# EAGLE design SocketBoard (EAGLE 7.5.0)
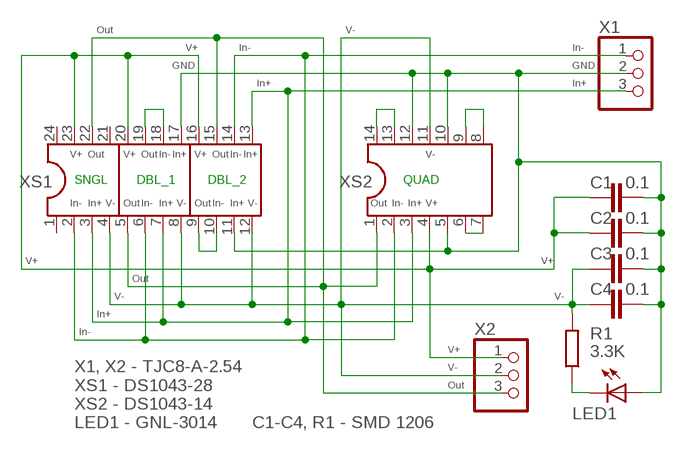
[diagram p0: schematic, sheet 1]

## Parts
C1  0.1  C-EUC1206  [C1206]
C2  0.1  C-EUC1206  [C1206]
C3  0.1  C-EUC1206  [C1206]
C4  0.1  C-EUC1206  [C1206]
LED1  GNL-3014  LED3MM  [LED3MM]
R1  3.3K  R-EU_R1206  [R1206]
X1  KF2510  PINHD-1X3  [1X03]
X2  KF2510  PINHD-1X3  [1X03]
XS1  DS1043-28  DIL24-3  [DIL24-3]
XS2  DS1043-14  DIL14  [DIL14]

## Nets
GND: C1.2 C2.2 C3.1 C4.1 LED1.A X1.2 XS1.11 XS1.17 XS2.5 XS2.10 XS2.12
IN+: X1.3 XS1.3 XS1.7 XS1.13 XS2.3
IN-: X1.1 XS1.2 XS1.6 XS1.14 XS2.2
N$1: XS1.9 XS1.10
N$2: XS1.18 XS1.19
N$3: XS2.13 XS2.14
N$4: XS2.8 XS2.9
N$5: XS2.6 XS2.7
N$8: LED1.K(C) R1.1
OUT: X2.3 XS1.5 XS1.15 XS1.22 XS2.1
V+: C1.1 C2.1 X2.1 XS1.16 XS1.20 XS1.23 XS2.4
V-: C3.2 C4.2 R1.2 X2.2 XS1.4 XS1.8 XS1.12 XS2.11
Unconnected: XS1.1 XS1.21 XS1.24

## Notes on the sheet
- Out | V-
- V+ | In- | In-
- GND | GND
- In+ | In+
- V+ | Out | V+ | Out | In- | In+ | V+ | Out | In- | In+ | V-
- SNGL | DBL_1 | DBL_2 | QUAD
- In- | In+ | V- | Out | In- | In+ | V- | Out | In- | In+ | V- | Out | In- | In+ | V+
- V+ | V+
- Out
- V- | V-
- In+
- In-
- V+
- V-
- Out
- X1, X2 - TJC8-A-2.54
  XS1 - DS1043-28
  XS2 - DS1043-14
  LED1 - GNL-3014
- C1-C4, R1 - SMD 1206

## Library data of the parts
C1-C4 = resistor:C-EU: CAPACITOR, European symbol
LED1 = led:LED: LED
R1 = resistor:R-EU_: RESISTOR, European symbol
X1 X2 = pinhead:PINHD-1X3: PIN HEADER
XS1 = ic-package:DIL24: Dual In Line
XS2 = ic-package:DIL14: Dual In Line / Socket

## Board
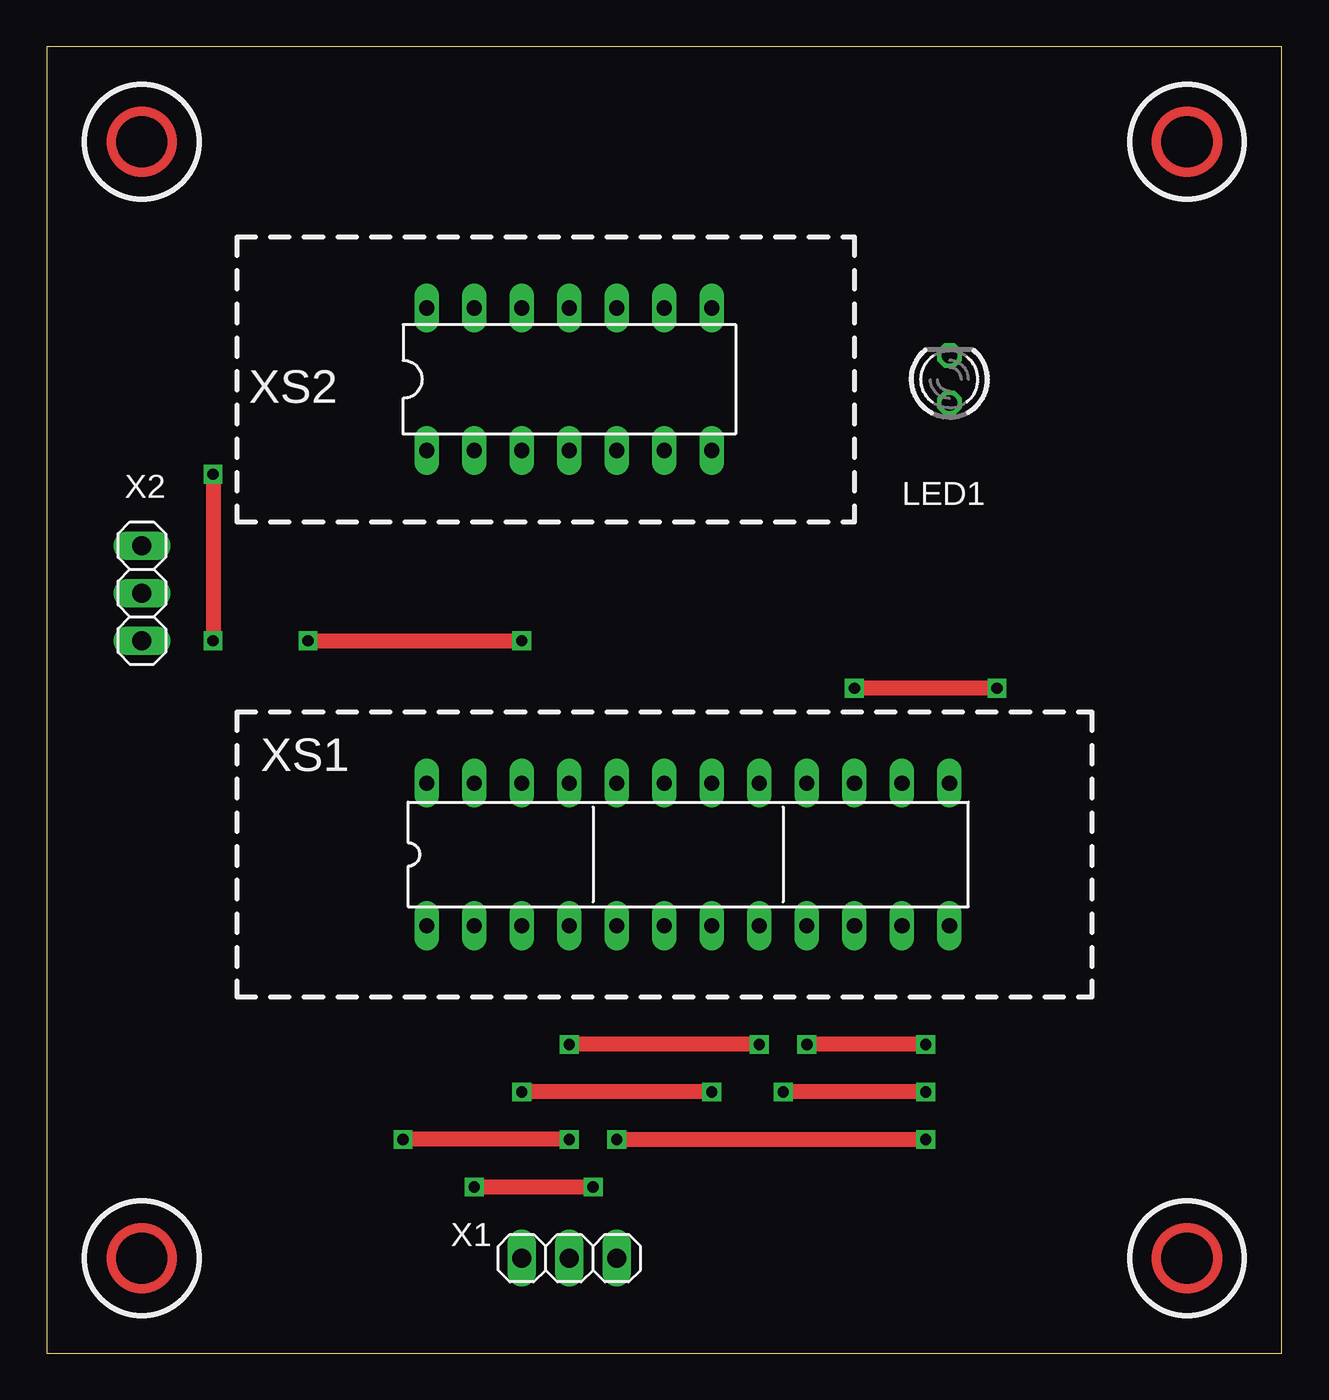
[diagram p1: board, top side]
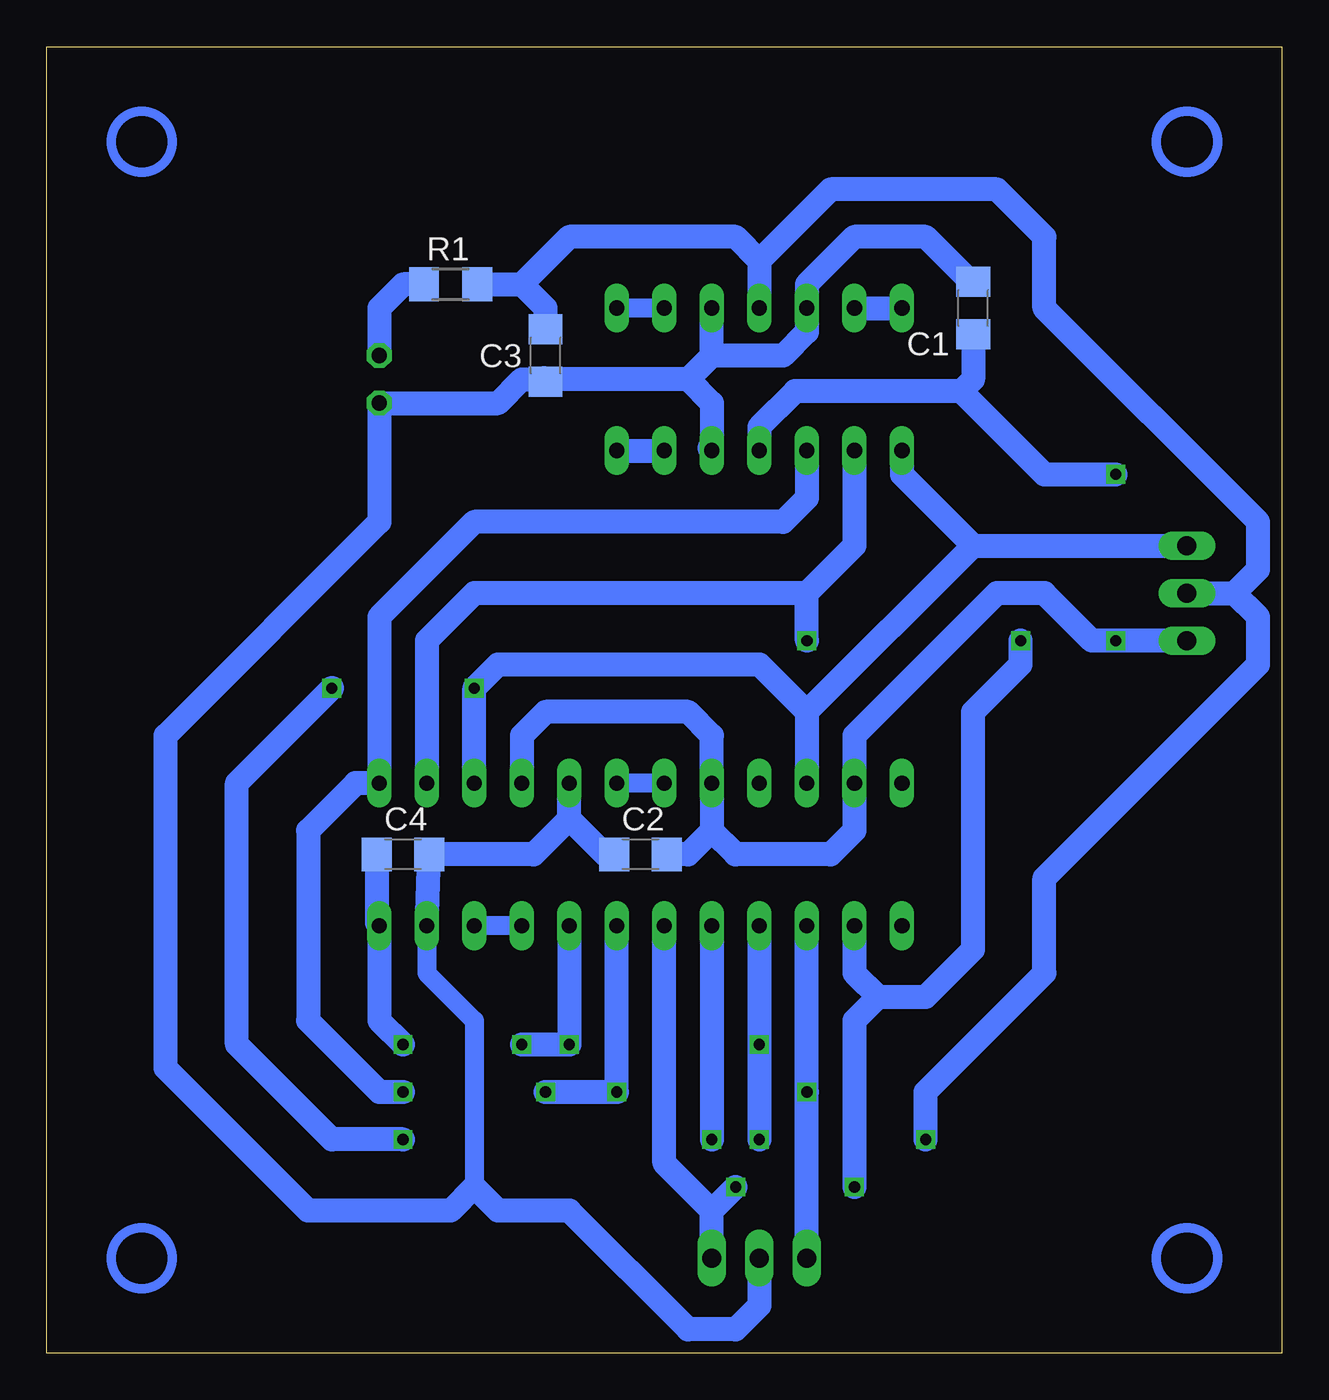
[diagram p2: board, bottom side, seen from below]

Size 66.04 x 69.85 mm. Coordinates in mm from the lower left corner, seen from the top.
Outline: 0,0 66.04,0 66.04,69.85 0,69.84 0,0
Copper layers (1*16): Top 0.035mm / dielectric 1.5mm / Bottom 0.035mm
Design rules "default *": minimum track width 10mil, minimum drill 24mil, track to track 8mil, track to pad 8mil, pad to pad 8mil, via to via 8mil, smd to smd 8mil, copper to edge 10mil, drill to drill 8mil, minimum pad ring 10mil, minimum via ring 8mil, stop-mask expansion 4mil, vias tented up to drill 0mil, thermal gap 10mil

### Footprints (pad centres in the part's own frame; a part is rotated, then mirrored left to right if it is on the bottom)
C1206 = smd 1.6 x 1.8: 1 -1.4,0; 2 1.4,0
LED3MM = drill 0.813 octagon: A -1.27,0; K 1.27,0
R1206 = smd 1.6 x 1.803: 1 -1.422,0; 2 1.422,0
1X03 = drill 1.016 long: 1 -2.54,0; 2 0,0; 3 2.54,0
DIL24-3 = drill 0.813 long: 1 -13.97,-3.81; 2 -11.43,-3.81; 3 -8.89,-3.81; 4 -6.35,-3.81; 5 -3.81,-3.81; 6 -1.27,-3.81; 7 1.27,-3.81; 8 3.81,-3.81; 9 6.35,-3.81; 10 8.89,-3.81; 11 11.43,-3.81; 12 13.97,-3.81; 13 13.97,3.81; 14 11.43,3.81; 15 8.89,3.81; 16 6.35,3.81; 17 3.81,3.81; 18 1.27,3.81; 19 -1.27,3.81; 20 -3.81,3.81; 21 -6.35,3.81; 22 -8.89,3.81; 23 -11.43,3.81; 24 -13.97,3.81
DIL14 = drill 0.813 long: 1 -7.62,-3.81; 2 -5.08,-3.81; 3 -2.54,-3.81; 4 0,-3.81; 5 2.54,-3.81; 6 5.08,-3.81; 7 7.62,-3.81; 8 7.62,3.81; 9 5.08,3.81; 10 2.54,3.81; 11 0,3.81; 12 -2.54,3.81; 13 -5.08,3.81; 14 -7.62,3.81

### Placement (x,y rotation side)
C1  16.51,55.88 90 bottom
C2  34.29,26.67 180 bottom
C3  39.37,53.34 90 bottom
C4  46.99,26.67 180 bottom
LED1  48.26,52.07 90 top
R1  44.45,57.15 0 bottom
X1  27.94,5.08 180 top
X2  5.08,40.64 90 top
XS1  34.29,26.67 0 top
XS2  27.94,52.07 0 top

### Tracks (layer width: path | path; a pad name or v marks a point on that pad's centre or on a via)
GND
  Bottom 1.016: 45.72,22.73 45.72,20.32 43.18,17.78 43.18,8.89
  Bottom 1.27: X1.2 27.94,2.54 29.21,1.27 31.75,1.27 38.1,7.62 41.91,7.62 43.18,8.89 44.45,7.62 52.07,7.62 59.69,15.24 59.69,33.02 48.26,44.45 LED1.A 41.91,50.8 40.64,52.07 39.5,52.07 39.45,52.13 | 30.61,48.39 XS2.5 30.48,50.8 31.75,52.07 | XS1.11 45.72,22.73 C4.1 40.01,26.67 38.1,28.57 | 38.1,28.57 XS1.17 | C2.2 36.2,26.67 38.1,28.57 | 39.45,52.13 C3.1 | 30.48,53.34 26.67,53.34 25.4,54.61 XS2.12 25.4,57.15 22.86,59.69 19.05,59.69 16.64,57.28 C1.2 | 31.75,52.07 39.39,52.07 39.45,52.13 | 30.48,53.34 XS2.10 | 31.75,52.07 30.48,53.34
IN+  (via drill 0.6)
  Top 0.813: v46.99,13.97 v39.37,13.97 | v35.56,13.97 v25.4,13.97
  Bottom 1.27: X1.3 v25.4,13.97 XS1.3 | v46.99,13.97 48.26,13.97 52.07,17.78 52.07,27.94 49.53,30.48 XS1.13 48.26,39.37 43.18,44.45 26.67,44.45 25.4,45.72 XS2.3 | v39.37,13.97 v35.56,13.97 XS1.7
IN-  (via drill 0.6)
  Top 0.813: v22.86,8.89 v29.21,8.89 | v13.97,38.1 v25.4,38.1
  Bottom 1.27: X1.1 30.48,7.62 | 30.48,7.62 33.02,10.16 XS1.6 | XS1.2 22.86,20.32 21.59,19.05 | 21.59,19.05 22.86,17.78 v22.86,8.89 | v29.21,8.89 30.48,7.62 | XS2.2 22.86,43.18 25.4,40.64 | 25.4,40.64 43.18,40.64 45.72,38.1 XS1.14 | 21.59,19.05 19.05,19.05 16.51,21.59 16.51,34.29 13.97,36.83 v13.97,38.1 | v25.4,38.1 25.4,40.64
N$1
  Bottom 1.016: XS1.9 XS1.10
N$2
  Bottom 1.016: XS1.19 XS1.18
N$3
  Bottom 1.27: XS2.13 XS2.14
N$4
  Bottom 1.016: XS2.9 XS2.8
N$5
  Bottom 1.27: XS2.7 XS2.6
N$8
  Bottom 1.27: R1.1 46.99,57.15 48.26,55.88 LED1.K
OUT  (via drill 0.6)
  Top 0.813: v30.48,11.43 v46.99,11.43 | v50.8,35.56 v43.18,35.56
  Bottom 1.27: XS2.1 20.32,46.99 16.51,43.18 | 16.51,43.18 X2.3 | 16.51,43.18 25.4,34.29 | 25.4,34.29 XS1.22 | XS1.15 v43.18,35.56 41.91,36.83 27.94,36.83 25.4,34.29 | XS1.5 v30.48,11.43 | v46.99,11.43 50.8,11.43 55.88,16.51 55.88,30.48 v50.8,35.56
V+  (via drill 0.6)
  Top 0.813: v8.89,46.99 v8.89,38.1
  Bottom 1.27: C1.1 16.51,52.07 17.14,51.44 | 17.14,51.44 26.04,51.44 27.94,49.53 XS2.4 | 30.48,27.94 XS1.20 30.48,33.02 31.75,34.29 39.37,34.29 40.64,33.02 XS1.16 | 30.48,27.94 31.75,26.67 C2.1 | 30.48,27.94 29.21,26.67 24.13,26.67 22.86,27.94 XS1.23 22.86,33.02 15.24,40.64 12.7,40.64 10.16,38.1 v8.89,38.1 X2.1 | 17.14,51.44 12.7,46.99 v8.89,46.99
V-  (via drill 0.6)
  Top 0.813: v27.94,11.43 v19.05,11.43 | v38.1,16.51 v27.94,16.51 | v46.99,16.51 v40.64,16.51
  Bottom 1.27: C4.2 48.39,22.99 XS1.12 48.26,17.78 v46.99,16.51 | X2.2 2.54,40.64 | 2.54,40.64 1.27,41.91 1.27,44.45 12.7,55.88 12.7,59.69 15.24,62.23 24.13,62.23 27.94,58.42 | 27.94,58.42 XS2.11 | XS1.4 v27.94,16.51 v27.94,11.43 | v19.05,11.43 19.05,13.97 12.7,20.32 12.7,25.4 1.27,36.83 1.27,39.37 2.54,40.64 | C3.2 39.37,55.88 40.64,57.15 | R1.2 40.64,57.15 | 27.94,58.42 29.21,59.69 38.1,59.69 40.64,57.15 | XS1.8 v38.1,16.51 v40.64,16.51
(copper drawn outside any net)
  shapes: Bottom circle x4, Top circle x4

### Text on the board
tDocu: Out | V- | V+ | In+ | GND | In-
